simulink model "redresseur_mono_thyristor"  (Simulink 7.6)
settings: Solver=ode23tb  StartTime=0.0  StopTime=0.04  RelTol=1e-4
StopFcn:
  | delete *.mat
libraries: powerlib x6, powerlib_extras x1

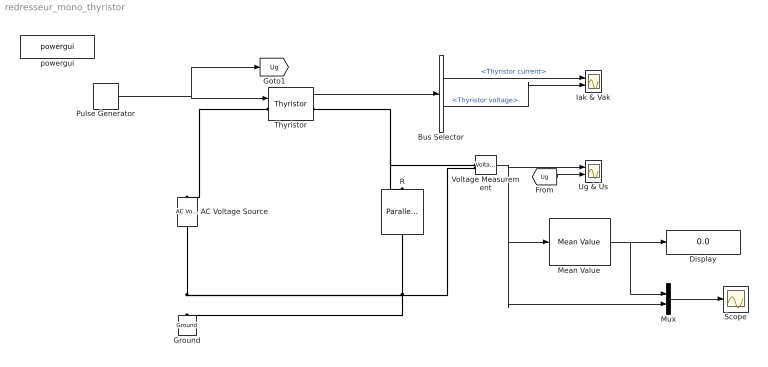
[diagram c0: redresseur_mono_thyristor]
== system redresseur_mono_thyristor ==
  AC Voltage Source : powerlib/Electrical Sources/AC Voltage Source  DialogController=POWERSYS.PowerSysDialog  SystemSampleTime=-1  Amplitude=100  Phase=0  Frequency=60  SampleTime=0  Measurements=None
  Bus Selector : BusSelector  OutputSignals=Thyristor current,Thyristor voltage
  Display : Display
  Ground : powerlib/Elements/Ground  DialogController=POWERSYS.PowerSysDialog  PhysicalDomain=powersysdomain  SubClassName=unknown  LeftPortType=p1  RightPortType=p1  LConnTagsString=a
  Iak & Vak : Scope  NumInputPorts=2
  Mean Value : powerlib_extras/Measurements/Mean Value  DialogController=POWERSYS.PowerSysDialog  SystemSampleTime=-1  Period=1/60
  Mux : Mux  Inputs=2
  Pulse Generator : DiscretePulseGenerator  PulseType=Time based  Period=1/120  PulseWidth=2  PhaseDelay=0.2/120
  R : powerlib/Elements/Parallel RLC Branch  DialogController=POWERSYS.PowerSysDialog  PhysicalDomain=powersysdomain  SubClassName=unknown  LeftPortType=p1  RightPortType=p1  LConnTagsString=a  RConnTagsString=__new0  BranchType=R  Resistance=1  Inductance=1e-3  SetiL0=off  InitialCurrent=0  Capacitance=1e-6  Setx0=off  InitialVoltage=0  Measurements=None
  Scope : Scope
  Thyristor : powerlib/Power Electronics/Thyristor  DialogController=POWERSYS.PowerSysDialog  SystemSampleTime=-1  Ron=0.001  Lon=0  Vf=0.8  IC=0  Rs=500  Cs=250e-9  Measurements=on
  Ug & Us : Scope  NumInputPorts=2
  Voltage Measurement : powerlib/Measurements/Voltage Measurement  DialogController=POWERSYS.PowerSysDialog  SystemSampleTime=-1  PhasorSimulation=off  OutputType=Complex  PSBequivalent=0
  powergui : powerlib/powergui  Priority=2  SystemSampleTime=-1  SimulationMode=Continuous  SampleTime=0  frequency=60  SPID=off  DisableSnubberDevices=off  DisableRonSwitches=off  DisableVfSwitches=off  SwTol=0  Interpol=off  frequencyindice=0  echomessages=off  HookPort=off  DisplayEquations=off  FunctionMessages=off  EnableUseOfTLC=off  x0status=blocks  RestoreLinks=warning  ResistiveCurrentMeasurement=off  Frange=logspace(0,3,50)  Ylog=off  Xlog=off  ShowGrid=off  save=off  variable=ZData  ZoomFFT=on  StartTime=0.0  cycles=1  DisplayStyle=off  fundamental=60  FreqAxis=off  MaxFrequency=1000  frequencyindicesteady=1  RmsSteady=1  display=off  Ts=0  methode=off
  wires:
  Bus Selector/1 -> Iak & Vak/1  "<Thyristor current>"
  Bus Selector/2 -> Iak & Vak/2  "<Thyristor voltage>"
  Thyristor/1 -> Bus Selector/1
  Pulse Generator/1 -> Thyristor/1, [Ug]
  Voltage Measurement/1 -> Ug & Us/1, Mean Value/1, Mux/2
  [Ug] -> Ug & Us/2
  Mean Value/1 -> Display/1, Mux/1
  Mux/1 -> Scope/1
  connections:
  AC Voltage Source/LConn1 -- Ground/LConn1 -- R/RConn1 -- Voltage Measurement/LConn2
  Thyristor/LConn1 -- AC Voltage Source/RConn1
  Thyristor/RConn1 -- R/LConn1 -- Voltage Measurement/LConn1
